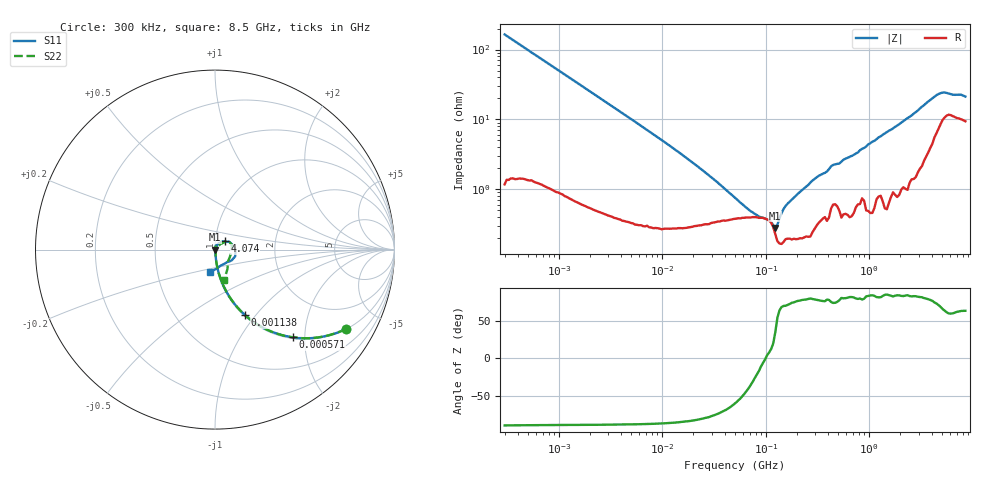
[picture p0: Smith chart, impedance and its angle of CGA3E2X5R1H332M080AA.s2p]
! S-parameter Generated by TDK Corporation
! Copyright(C) 2015 TDK Corporation.
! All Rights Reserved.
! TDK P/N: CGA3E2X5R1H332M080AA (Multilayer Ceramic Chip Capacitors)
! Property: C=3.3nF
! Size(LxWxT): 1.6x0.8x0.8mm, 0.063x0.031x0.031inches
! Model Type: s2p (Touchstone File Format Version 1.0)
! Frequency: DC=Yes Start=0.3MHz Stop=8500MHz 225points Log-sweep
! Note:
! Model Generated on Jun. 23, 2015
! Hash(MD5):
! Port Assignments:
!  1 ---| |--- 2
! Applicable Conditions:
!  Temperature = 25 degC
!  DC Bias Voltage = 0 V
!  Small Signal Operation
! Terms and conditions regarding TDK Simulation Models
! (1)This simulation model is being provided solely for informational purposes. Please refer to the specifications of the products in terms of detailed characteristics of such products.
! (2)In no event shall TDK Corporation of any of its subsidiaries be liable for any loss or damage arising, directly or indirectly,
!  From any information contained in this simulation model, including, but not limited to loss or damages arising from any inaccuracies, omissions or errors in connection with such information.
! (3)Any and all copyrights on this simulation model are owned by TDK Corporation.
!  Duplication or redistribution of this simulation model without prior written permission from TDK Corporation is prohibited.
! (4)This simulation model is subject to any modification or change without any prior notice.
! (5)Neither TDK Corporation nor any of its subsidiaries shall make any warranty, express or implied,
!  Including but not limited to the correctness, implied warranties of merchantability and fitness for a particular purpose with respect to this simulation models.
! (6)The use of this simulation model shall be deemed to have consented to the terms and conditions hereof.
# MHz S MA R 50
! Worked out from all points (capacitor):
!   224 points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, 300 kHz to 8.5 GHz, reference 50 ohm
!   read as one part in series: C = 3.21 nF near 314.1 kHz
!   lowest |Z| = 278 mohm at 123.8 MHz (marker M1)
!   series resonance near 99.64 MHz, so ESL is about 790 pH
!   S11 on the Smith chart (normalised r, x): 300 kHz: 1.01, -3.30; 571 kHz: 1.02, -1.74; 1.138 MHz: 1.01, -0.88; 4.074 GHz: 1.11, +0.10; 8.5 GHz: 0.92, -0.24
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0.3  0.8536 -31.2  0.518 58.4  0.5171 58.8  0.8531 -31.2
0.5710021  0.6526 -48.5  0.7488 40.7  0.7469 40.9  0.6526 -48.5
1.137941  0.4013 -65.4  0.9103 23.6  0.9082 23.8  0.4013 -65.4
1.72111  0.2798 -72.7  0.9559 16.2  0.9539 16.4  0.2796 -72.7
9.430415  0.05333 -84.3  0.9968 2.9  0.9951 3.1  0.05308 -84.2
51.67171  0.007997 -69.7  0.9968 0.1  0.9952 0.4  0.01003 -64.7
123.7646  0.002104 -18.6  0.9973 -0.4  0.9957 -0.2  0.004317 -88.8
142.0669  0.0006796 -129.5  0.9981 -0.7  0.9965 -0.4  0.002498 -51.3
170.7477  0.00176 158.9  0.9966 -0.9  0.995 -0.6  0.002145 -58.9
205.2186  0.002108 155.2  0.9958 -1.1  0.9942 -0.8  0.0005523 -131.6
283.1228  0.001825 136.0  0.995 -1.5  0.9934 -1.2  0.004165 97.2
340.2802  0.0008011 51.1  0.9941 -1.7  0.9926 -1.5  0.006691 84.8
448.3627  0.007665 48.1  0.9936 -2.2  0.9921 -2.0  0.007611 47.8
514.6664  0.008184 64.7  0.9935 -2.5  0.9919 -2.2  0.003166 49.3
618.5683  0.007255 94.1  0.9919 -3.0  0.9906 -2.7  0.004041 75.9
743.4462  0.002345 48.8  0.9914 -3.5  0.99 -3.2  0.009477 73.6
893.5346  0.01127 53.5  0.9919 -4.1  0.9907 -3.8  0.006914 51.1
1124.446  0.006231 76.5  0.991 -5.3  0.9895 -5.0  0.0116 75.6
1290.729  0.01571 58.6  0.99 -5.9  0.9889 -5.6  0.0117 59.8
1551.304  0.01304 79.1  0.9893 -7.1  0.9877 -6.9  0.01605 74.4
4073.536  0.07113 40.7  0.9506 -19.2  0.9476 -18.6  0.07716 36.5
8500  0.1299 -102.5  0.887 -31.6  0.8865 -30.8  0.1753 -72.5
